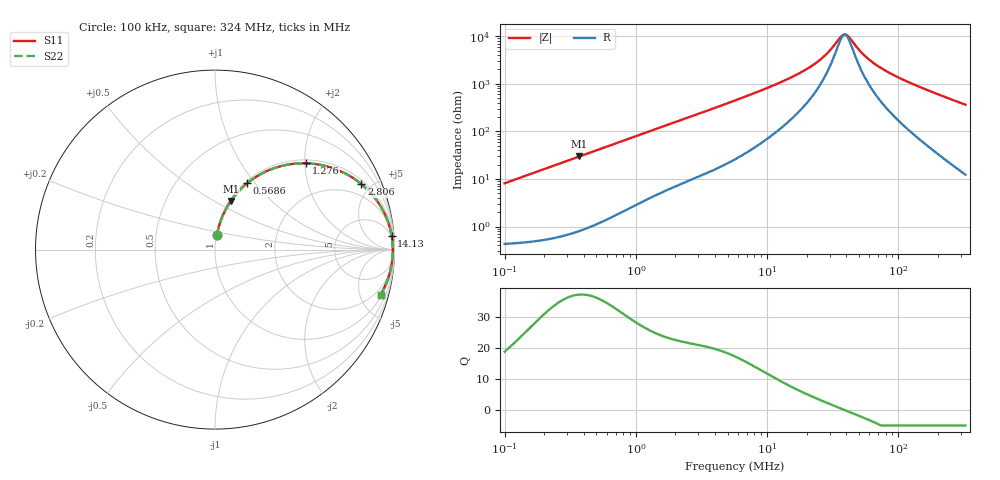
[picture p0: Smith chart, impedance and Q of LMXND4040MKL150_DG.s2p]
! LMXND4040MKL150_DG  S-PARAMETER MODEL  ( General Type )
! Model Generated by TAIYO YUDEN Corporation (http://www.ty-top.com)
! Version 1.0
! TAIYO YUDEN Control No. 191023NI43SB-FBB
! Copyright(c) 2019 TAIYO YUDEN CO.,LTD. All Rights Reserved.
! Product Description (link to TY-COMPAS)
! https://ds.yuden.co.jp/TYCOMPAS/or/detail?pn=LMXND4040MKL150MDG&u=M
! Products Name : Inductors
! Characteristics :
!  Inductance : 15 uH , SRF(min) : 24 MHz , DC Resistance(max) : 0.312 Ohm
!  Rated Current : Saturation :650 mA , Temp Rise : 750 mA
!  Case Size : 4.0 x 4.0 / 0.157 x 0.157 [mm/inch] , Thickness : 1.2 / 0.047 [mm/inch]
!  (Conditions: Temperature = 25 degC , DC Bias Current/Voltage = 0A / 0V)
! External Node Assignments :
!  1  o---GGG---o  2
! GND o---------o GND
! Frequency Range : 0.1MHz  -  324.04089MHz  [ 402 STEP ]
# MHz S RI R 50
! Freq[MHz].  S11 Real  S11 Imag  S21 Real  S21 Imag  S12 Real  S12 Imag  S22 Real  S22 Imag
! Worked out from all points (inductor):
!   401 points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, 100 kHz to 324 MHz, reference 50 ohm
!   read as one part in series: L = 12.9 uH near 104.1 kHz
!   highest Q = 37.2 at 371.9 kHz (marker M1), where L = 12.8 uH
!   self-resonance near 38.82 MHz
!   S11 on the Smith chart (normalised r, x): 100 kHz: 1.01, +0.16; 568.6 kHz: 1.03, +0.91; 1.276 MHz: 1.08, +2.02; 2.806 MHz: 1.21, +4.37; 14.13 MHz: 4, +25; 324 MHz: 1.25, -7.27
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0.1  0.0107 0.0797  0.9893 -0.0797  0.9893 -0.0797  0.0107 0.0797
0.198793  0.0299 0.1547  0.9701 -0.1547  0.9701 -0.1547  0.0299 0.1547
0.37194  0.0884 0.2707  0.9116 -0.2707  0.9116 -0.2707  0.0884 0.2707
0.38728  0.0948 0.2798  0.9052 -0.2798  0.9052 -0.2798  0.0948 0.2798
0.568563  0.1794 0.3697  0.8206 -0.3697  0.8206 -0.3697  0.1794 0.3697
0.886874  0.3392 0.4569  0.6608 -0.4569  0.6608 -0.4569  0.3392 0.4569
1.275966  0.5057 0.4809  0.4943 -0.4809  0.4943 -0.4809  0.5057 0.4809
1.499861  0.5807 0.4733  0.4193 -0.4733  0.4193 -0.4733  0.5807 0.4733
2.806225  0.8159 0.3647  0.1841 -0.3647  0.1841 -0.3647  0.8159 0.3647
5.692459  0.9412 0.2081  0.0588 -0.2081  0.0588 -0.2081  0.9412 0.2081
14.13326  0.9841 0.0784  0.0159 -0.0784  0.0159 -0.0784  0.9841 0.0784
22.04577  0.9891 0.0396  0.0109 -0.0396  0.0109 -0.0396  0.9891 0.0396
28.09593  0.9903 0.022  0.00967 -0.022  0.00967 -0.022  0.9903 0.022
36.53742  0.9909 0.00432  0.00913 -0.00432  0.00913 -0.00432  0.9909 0.00432
39.61356  0.9909 -0.00101  0.00909 0.00101  0.00909 0.00101  0.9909 -0.00101
42.08946  0.9909 -0.00501  0.00911 0.00501  0.00911 0.00501  0.9909 -0.00501
50.48494  0.9906 -0.0172  0.00936 0.0172  0.00936 0.0172  0.9906 -0.0172
58.15638  0.9902 -0.027  0.00979 0.027  0.00979 0.027  0.9902 -0.027
69.75669  0.9893 -0.0405  0.0107 0.0405  0.0107 0.0405  0.9893 -0.0405
85.37896  0.9877 -0.0569  0.0123 0.0569  0.0123 0.0569  0.9877 -0.0569
150.3463  0.977 -0.1169  0.023 0.1169  0.023 0.1169  0.977 -0.1169
324.0409  0.9224 -0.2512  0.0776 0.2512  0.0776 0.2512  0.9224 -0.2512
